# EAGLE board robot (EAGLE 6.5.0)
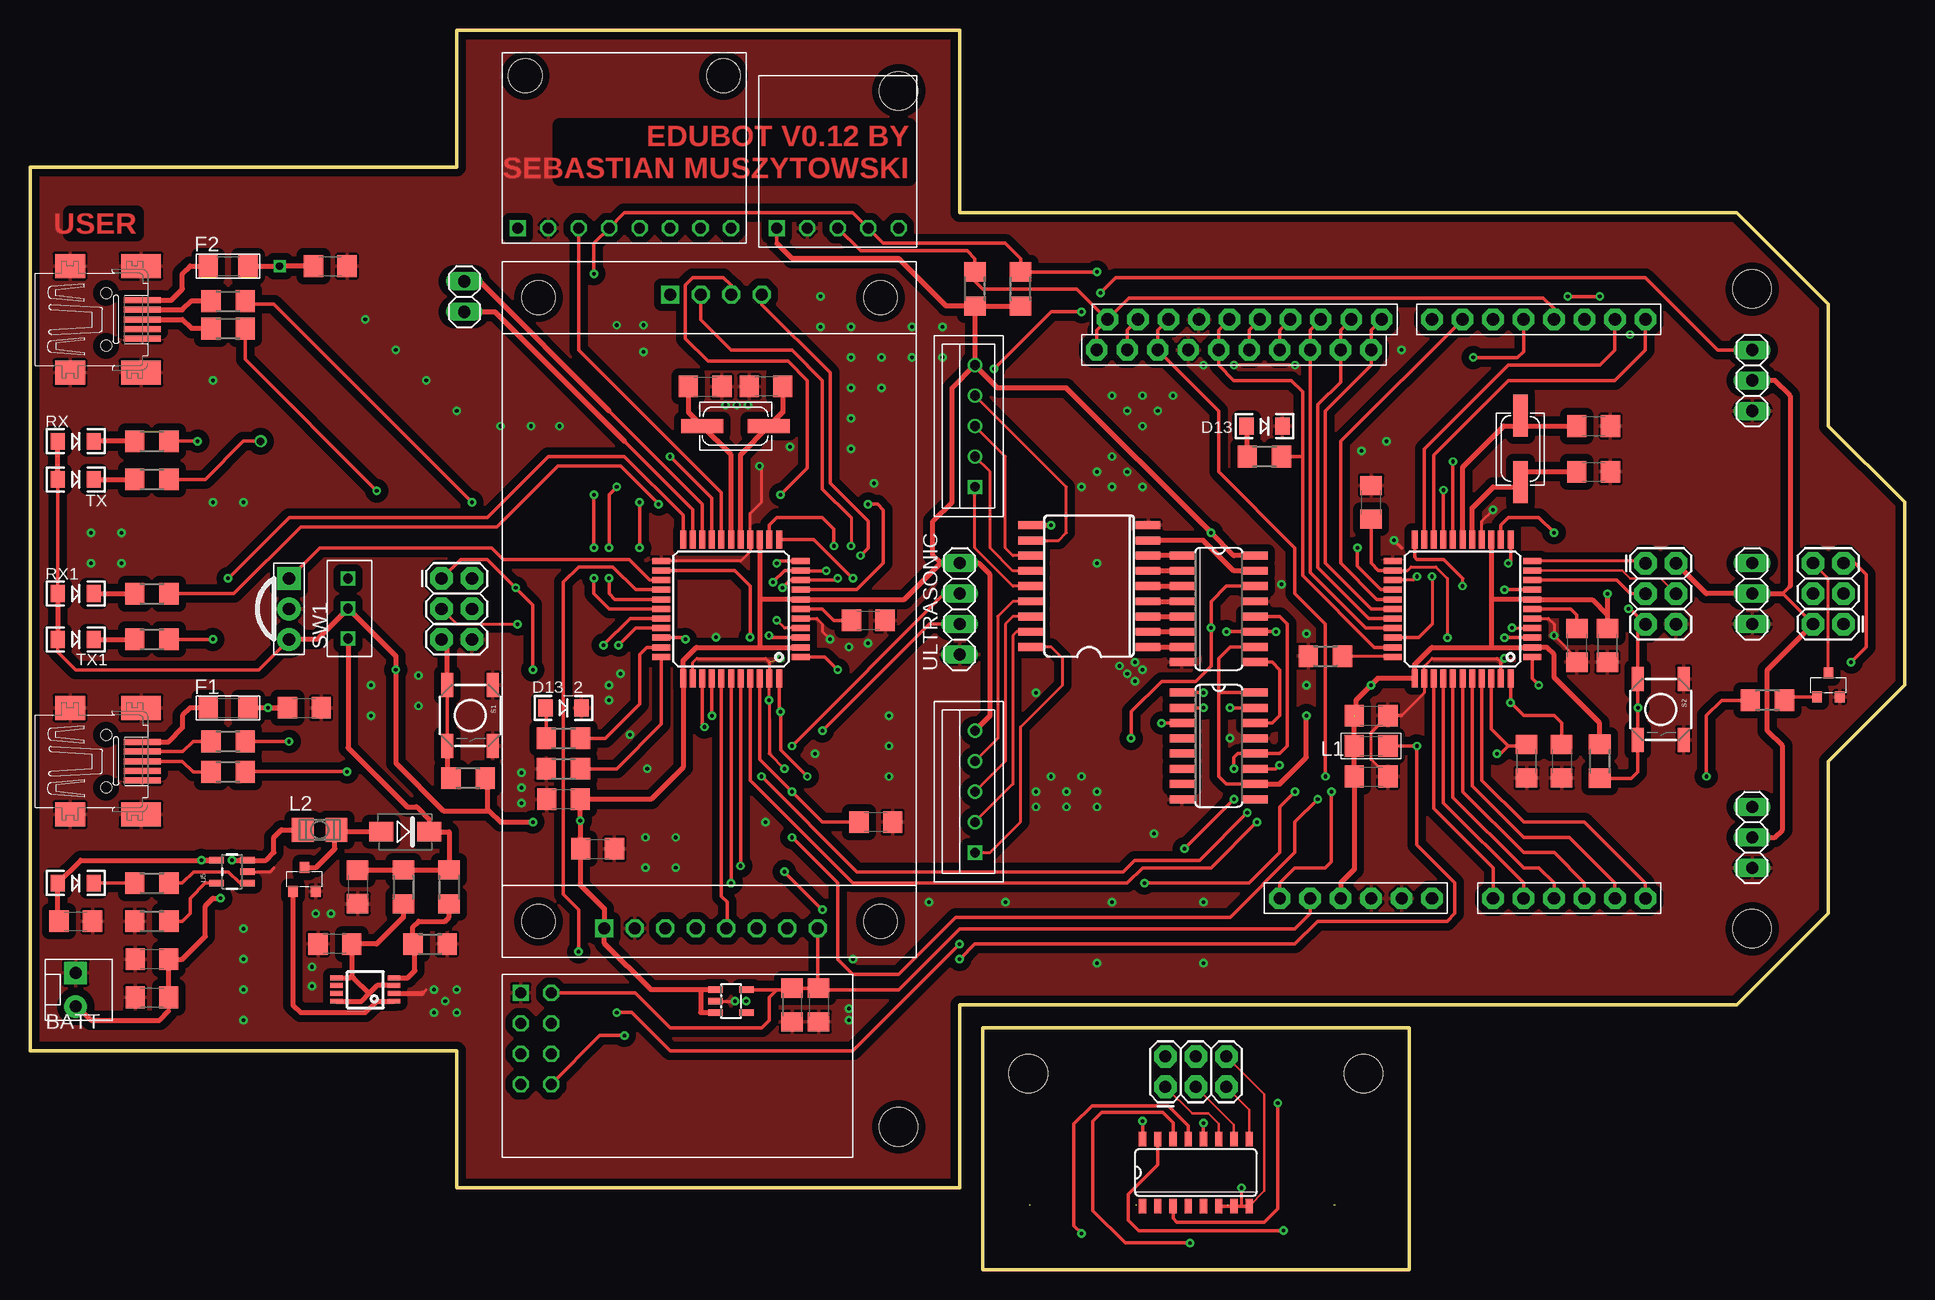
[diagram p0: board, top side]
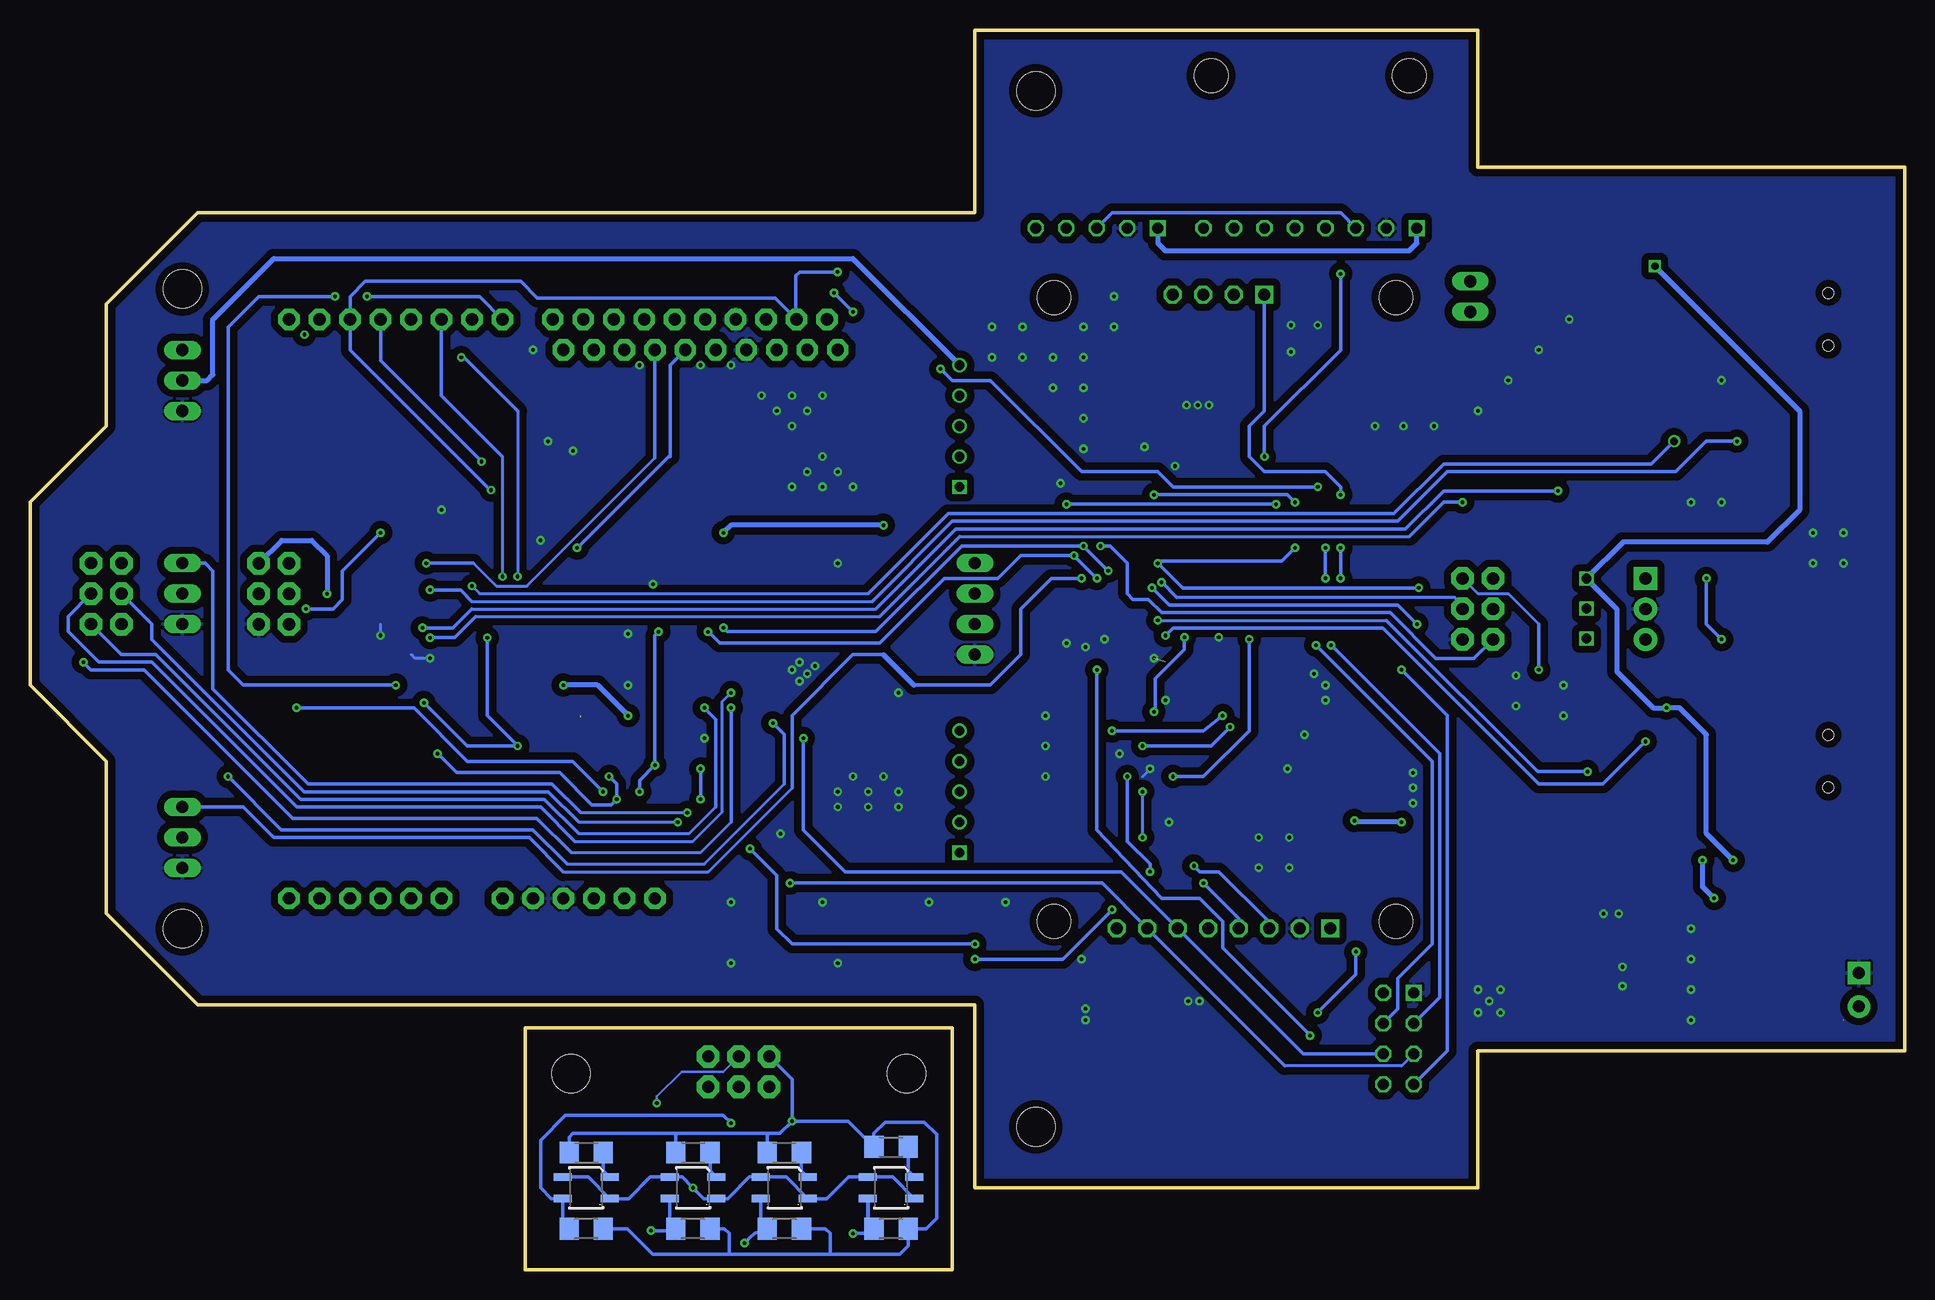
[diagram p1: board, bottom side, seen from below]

Size 156.21 x 103.35 mm. Coordinates in mm from the lower left corner, seen from the top.
Outline: 79.38,20.16 114.94,20.16 114.94,0 79.38,0 79.38,20.16
Outline: 156.21,48.74 149.86,42.39 149.86,29.69 142.24,22.07 77.47,22.07 77.47,6.83 35.56,6.83 35.56,18.26 0,18.26 0,91.92 35.56,91.92 35.56,103.35 77.47,103.35 77.47,88.11 142.24,88.11 149.86,80.49 149.86,70.33 156.21,63.98 156.21,48.74
Copper layers (1*16): Top 0.035mm / dielectric 1.5mm / Bottom 0.035mm
Design rules "pcb-devboards_35µmCU_200µm_Strukturen_Abstaende": minimum track width 0.2mm, minimum drill 0.3mm, track to track 0.2mm, track to pad 0.2mm, pad to pad 0.2mm, via to via 0.2mm, smd to smd 0.2mm, copper to edge 0.4mm, drill to drill 0.4mm, minimum pad ring 0.2mm, minimum via ring 0.2mm, stop-mask expansion 4mil, vias tented up to drill 0mil, thermal gap 0.2mm
Net classes: 1 vcc: width 0.254 mm
Holes 3.2 mm at 83.19,16.35 111.12,16.35 72.39,11.91 72.39,98.27 143.51,81.76 143.51,28.42

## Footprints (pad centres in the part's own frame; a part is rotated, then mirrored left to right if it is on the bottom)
MOLEX-1X2_LOCK = drill 1.016 pad 1.88 square: 1 -0.127,0 | drill 1.016 pad 1.88: 2 2.667,0
C1206 = smd 1.6 x 1.8: 1 -1.4,0; 2 1.4,0
1X06-BIG = drill 1.016 pad 1.778 octagon: 1 -6.35,0; 2 -3.81,0; 3 -1.27,0; 4 1.27,0; 5 3.81,0; 6 6.35,0
1X08-BIG = drill 1.016 pad 1.778 octagon: 1 -8.89,0; 2 -6.35,0; 3 -3.81,0; 4 -1.27,0; 5 1.27,0; 6 3.81,0; 7 6.35,0; 8 8.89,0
1X10-BIG = drill 1.016 pad 1.778 octagon: 1 -11.43,0; 2 -8.89,0; 3 -6.35,0; 4 -3.81,0; 5 -1.27,0; 6 1.27,0; 7 3.81,0; 8 6.35,0; 9 8.89,0; 10 11.43,0
SMA = smd 2 x 1.65: A 5,0.8; C 1,0.8
LED-1206 = smd 1.2 x 1.4: A -1.5,0; C 1.5,0
1206_PTC = smd 1.6 x 1.8: 1 -1.654,0; 2 1.654,0
MICRO3 = smd 0.8 x 0.9: 1 -0.95,-1; 2 0.95,-1; 3 0,1
2X3 = drill 1.016 pad 1.88 octagon: 1 0,0; 2 0,2.54; 3 2.54,0; 4 2.54,2.54; 5 5.08,0; 6 5.08,2.54
1206W = smd 1.6 x 1.8: 1 -1.4,0; 2 1.4,0
L3225P = smd 1.8 x 2: 1 -1.4,0; 2 1.4,0
32005-201 = smd 3.1 x 0.5: 1 3,1.6; 2 3,0.8; 3 3,0; 4 3,-0.8; 5 3,-1.6 | smd 2.5 x 2: M1 -3,-4.45; M2 -3,4.45 | smd 3.3 x 2: M3 2.9,4.45; M4 2.9,-4.45 | hole 0.9: 0,2.2; 0,-2.2
SO16 = smd 0.6 x 1.2: 1 -4.445,-2.8; 2 -3.175,-2.8; 3 -1.905,-2.8; 4 -0.635,-2.8; 5 0.635,-2.8; 6 1.905,-2.8; 7 3.175,-2.8; 8 4.445,-2.8; 9 4.445,2.8; 10 3.175,2.8; 11 1.905,2.8; 12 0.635,2.8; 13 -0.635,2.8; 14 -1.905,2.8; 15 -3.175,2.8; 16 -4.445,2.8
CSM-3X = smd 3.5 x 1.2: 1 2.775,0; 2 -2.775,0
QRE1113 = smd 1.5 x 0.6: 1 -1.95,-0.9; 2 1.95,-0.9; 3 1.95,0.9; 4 -1.95,0.9
R1206 = smd 1.6 x 1.803: 1 -1.422,0; 2 1.422,0
TACTILE_SWITCH_SMD = smd 2 x 1: 1 -2.54,1.905; 2 2.54,1.905; 3 -2.54,-1.905; 4 2.54,-1.905
1X02 = drill 1.016 long: 1 -1.27,0; 2 1.27,0
1X03 = drill 1.016 long: 1 -2.54,0; 2 0,0; 3 2.54,0
SO16' = smd 0.66 x 2.032: 1 -4.445,-3.073; 2 -3.175,-3.073; 3 -1.905,-3.073; 4 -0.635,-3.073; 5 0.635,-3.073; 6 1.905,-3.073; 7 3.175,-3.073; 8 4.445,-3.073; 9 4.445,3.073; 10 3.175,3.073; 11 1.905,3.073; 12 0.635,3.073; 13 -0.635,3.073; 14 -1.905,3.073; 15 -3.175,3.073; 16 -4.445,3.073
SO18L = smd 0.66 x 2.032: 1 -0.635,-4.902; 2 0.635,-4.902; 3 1.905,-4.902; 4 3.175,-4.902; 5 4.445,-4.902; 6 5.715,-4.902; 7 6.985,-4.902; 8 8.255,-4.902; 9 9.525,-4.902; 10 9.525,4.902; 11 8.255,4.902; 12 6.985,4.902; 13 5.715,4.902; 14 4.445,4.902; 15 3.175,4.902; 16 1.905,4.902; 17 0.635,4.902; 18 -0.635,4.902
SPDT-PTH = drill 0.8 square: 1 1.5,-1.75; 2 4,-1.75; 3 6.5,-1.75
TQFP44 = smd 1.5 x 0.5: 1 -5.8,4; 2 -5.8,3.2; 3 -5.8,2.4; 4 -5.8,1.6; 5 -5.8,0.8; 6 -5.8,0; 7 -5.8,-0.8; 8 -5.8,-1.6; 9 -5.8,-2.4; 10 -5.8,-3.2; 11 -5.8,-4; 23 5.8,-4; 24 5.8,-3.2; 25 5.8,-2.4; 26 5.8,-1.6; 27 5.8,-0.8; 28 5.8,0; 29 5.8,0.8; 30 5.8,1.6; 31 5.8,2.4; 32 5.8,3.2; 33 5.8,4 | smd 0.5 x 1.5: 12 -4,-5.8; 13 -3.2,-5.8; 14 -2.4,-5.8; 15 -1.6,-5.8; 16 -0.8,-5.8; 17 0,-5.8; 18 0.8,-5.8; 19 1.6,-5.8; 20 2.4,-5.8; 21 3.2,-5.8; 22 4,-5.8; 34 4,5.8; 35 3.2,5.8; 36 2.4,5.8; 37 1.6,5.8; 38 0.8,5.8; 39 0,5.8; 40 -0.8,5.8; 41 -1.6,5.8; 42 -2.4,5.8; 43 -3.2,5.8; 44 -4,5.8
SOT23-5@1 = smd 0.55 x 1.2: 1 -0.95,-1.3; 2 0,-1.3; 3 0.95,-1.3; 4 0.95,1.3; 5 -0.95,1.3
MSOP8 = smd 0.41 x 1.02: 1 -0.95,-2.4; 2 -0.3,-2.4; 3 0.35,-2.4; 4 1,-2.4; 5 1,2.4; 6 0.35,2.4; 7 -0.3,2.4; 8 -0.95,2.4
SOT23-5 = smd 0.55 x 1.2: 1 -0.95,-1.3; 2 0,-1.3; 3 0.95,-1.3; 4 0.95,1.3; 5 -0.95,1.3
1.8TFTSD = drill 1 square: P$1 55.58,8.5; P$9 2.76,14 | drill 1 octagon: P$2 55.58,11.04; P$3 55.58,13.58; P$4 55.58,16.12; P$5 55.58,18.66; P$6 55.58,21.2; P$7 55.58,23.74; P$8 55.58,26.28; P$10 2.76,16.54; P$11 2.76,19.08; P$12 2.76,21.62 | hole 2.8: 3,3; 3,31.5; 55,31.5; 55,3
GY-521 = drill 0.9 square: P$1 0,0 | drill 0.9 octagon: P$2 2.54,0; P$3 5.08,0; P$4 7.62,0; P$5 10.16,0; P$6 12.7,0; P$7 15.24,0; P$8 17.78,0 | hole 2.8: 0.635,12.7; 17.145,12.7
HMC5883L = drill 0.9 square: P$1 0,5.08 | drill 0.9 octagon: P$2 0,2.54; P$3 0,0; P$4 0,-2.54; P$5 0,-5.08
NRF24L01+ = drill 0.9 square: P$1 -1.016,1.016 | drill 0.9 octagon: P$2 -1.016,-1.524; P$3 -1.016,-4.064; P$4 -1.016,-6.604; P$5 1.524,-6.604; P$6 1.524,-4.064; P$7 1.524,-1.524; P$8 1.524,1.016
PNA460XM = drill 1.016 pad 1.93 square: 1 -2.54,0 | drill 1.016 pad 1.93: 2 0,0; 3 2.54,0
1X04 = drill 1.016 long: 1 -3.81,0; 2 -1.27,0; 3 1.27,0; 4 3.81,0
B5B-XH = drill 0.8 square: P$1 -5.08,0 | drill 0.8: P$2 -2.54,0; P$3 0,0; P$4 2.54,0; P$5 5.08,0

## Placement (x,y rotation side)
BATT  M02POLAR_LOCK  [MOLEX-1X2_LOCK]  3.81,24.61 270 top
C1  0.1uF  [C1206]  124.71,42.39 90 top
C2  0.1uF  [C1206]  44.45,39.21 180 top
C3  1uF  [C1206]  128.91,52.04 270 top
C4  1uF  [C1206]  131.44,52.04 270 top
C5  10uF  [C1206]  22.86,46.83 0 top
C6  10uF  [C1206]  25.02,83.66 0 top
C7  10uF  [C1206]  63.5,22.07 270 top
C8  0.1uF  [C1206]  70.48,37.31 180 top
C9  1uF  [C1206]  69.85,54.13 0 top
C10  0.1uF  [C1206]  111.76,46.2 0 top
C11  100nF  [C1206]  65.72,22.07 270 top
C12  1uF  [C1206]  111.76,41.12 0 top
C13  0.1uF  [C1206]  111.76,63.98 90 top
C14  0.1uF  [C1206]  127.64,42.39 270 top
C15  18pF  [C1206]  130.3,70.33 0 top
C16  18pF  [C1206]  130.3,66.52 0 top
C17  1uF  [C1206]  47.31,35.08 0 top
C18  47 uF  [C1206]  10.16,22.7 0 top
C19  0.1uF  [C1206]  25.4,27.15 180 top
C20  4.7uF  [C1206]  3.81,29.05 0 top
C21  4.7uF  [C1206]  10.16,25.88 180 top
C22  18pF  [C1206]  56.26,73.63 0 top
C23  18pF  [C1206]  61.34,73.63 180 top
C24  47 uF  [C1206]  27.3,31.91 270 top
CONN1  ANALOG  [1X06-BIG]  128.27,30.96 0 top
CONN2  DIGITAL  [1X08-BIG]  125.73,79.22 180 top
CONN3  DIGITAL  [1X10-BIG]  101.22,79.22 180 top
CONN4  DIGITAL RASTER  [1X10-BIG]  100.33,76.68 180 top
CONN5  POWER  [1X06-BIG]  110.49,30.96 0 top
D3  B330A  [SMA]  34.29,37.31 180 top
D4  POWER  [LED-1206]  3.81,32.23 0 top
D13  Green  [LED-1206]  102.87,70.33 0 top
D13_2  Green  [LED-1206]  44.45,46.83 0 top
F1  1206L  [1206_PTC]  16.51,46.83 0 top
F2  1206L  [1206_PTC]  16.51,83.66 0 top
FET1  TR  [MICRO3]  149.86,48.74 0 top
FET3  TR  [MICRO3]  22.86,32.54 0 top
JP1  ISP  [2X3]  34.29,57.63 270 top
JP2  [2X3]  151.13,53.82 90 top
JP3  ISP  [2X3]  134.62,58.89 270 top
JP4  [2X3]  94.61,15.24 0 top
L1  Ferrite  [1206W]  111.76,43.66 0 top
L2  BRL3225T3R3M  [L3225P]  24.13,36.67 0 top
MINIUSB  MINI-USB-SCHIELD-32005-201  [32005-201]  6.35,79.22 0 top
MINIUSB1  MINI-USB-SCHIELD-32005-201  [32005-201]  6.35,42.39 0 top
MUX  74HC4051  [SO16]  97.16,8.1 0 top
Q1  CSM-3X-CRYSTALCSM-3X  [CSM-3X]  124.21,68.42 90 top
Q2  QRE1113  [QRE1113]  84.45,6.83 180 bottom
Q3  QRE1113  [QRE1113]  93.34,6.83 180 bottom
Q4  QRE1113  [QRE1113]  100.97,6.83 180 bottom
Q5  QRE1113  [QRE1113]  109.86,6.83 180 bottom
Q6  CSM-3X-CRYSTALCSM-3X  [CSM-3X]  58.8,70.33 180 top
R1  100  [R1206]  84.45,10.24 180 bottom
R2  10K  [R1206]  130.81,42.39 90 top
R3  10K  [R1206]  84.45,3.41 0 bottom
R4  22  [R1206]  16.51,78.45 180 top
R5  22  [R1206]  16.51,80.74 180 top
R6  1K  [R1206]  102.87,67.79 180 top
R7  1K  [R1206]  10.16,69.06 180 top
R8  1K  [R1206]  10.16,65.88 180 top
R9  10K  [R1206]  107.95,51.15 180 top
R10  100  [R1206]  93.34,9.76 180 bottom
R11  10K  [R1206]  93.34,3.41 0 bottom
R12  100  [R1206]  100.97,9.76 180 bottom
R13  10K  [R1206]  100.97,3.41 0 bottom
R14  100  [R1206]  109.86,9.76 180 bottom
R15  10K  [R1206]  109.86,3.41 0 bottom
R16  22  [R1206]  16.51,41.5 180 top
R17  470  [R1206]  10.16,32.23 180 top
R18  100  [R1206]  144.78,47.47 0 top
R19  2K  [R1206]  10.16,29.05 180 top
R20  1K  [R1206]  44.45,44.29 180 top
R21  1K  [R1206]  10.16,56.36 180 top
R22  1K  [R1206]  10.16,52.55 180 top
R23  10K  [R1206]  36.51,40.96 0 top
R24  10K  [R1206]  44.45,41.75 180 top
R25  22  [R1206]  16.51,44.04 180 top
R26  2.2K  [R1206]  78.74,81.76 270 top
R27  2.2K  [R1206]  82.55,81.76 270 top
R46  100  [R1206]  31.11,31.91 90 top
R49  3.09k  [R1206]  34.92,31.91 90 top
R51  1K  [R1206]  33.34,27.15 180 top
RX  Green  [LED-1206]  3.81,69.06 0 top
RX1  Green  [LED-1206]  3.81,56.36 0 top
S1  Reset  [TACTILE_SWITCH_SMD]  36.67,46.2 270 top
S2  Reset  [TACTILE_SWITCH_SMD]  135.89,46.7 270 top
SER_CPU2  SER2  [1X02]  36.2,81.12 90 top
SERVO1(USONIC)  USONIC  [1X03]  143.51,56.36 90 top
SERVO2(GRIP)  GRIPPER  [1X03]  143.51,74.14 90 top
SERVO3(GRIPROT)  ROTATE  [1X03]  143.51,36.04 90 top
SHIFT1  74HC595D  [SO16']  99.06,55.09 270 top
SHIFT2  74HC595D  [SO16']  99.06,43.66 270 top
STEPPER_DRIVER  ULN2803  [SO18L]  88.27,52.55 90 top
SW1  [SPDT-PTH]  24.77,51.12 90 top
TX  Green  [LED-1206]  3.81,65.88 0 top
TX1  Green  [LED-1206]  3.81,52.55 0 top
U1  USER  [TQFP44]  119.38,55.09 180 top
U2  BRAIN  [TQFP44]  58.42,55.09 180 top
U3  LP2985  [SOT23-5@1]  58.42,22.38 270 top
U4  MCP1650  [MSOP8]  27.94,23.34 90 top
U5  MCP73831  [SOT23-5]  16.83,33.18 90 top
U$2  1.8TFT+SD  [1.8TFTSD]  39.37,84.04 270 top
U$3  GY-521  [GY-521]  40.64,86.84 0 top
U$4  HMC5883L  [HMC5883L]  67.31,86.84 90 top
U$5  NRF24L01+  [NRF24L01+]  41.91,22.07 0 top
U$10  PNA460XM  [PNA460XM]  21.59,55.09 270 top
ULTRASONIC  [1X04]  77.47,55.09 90 top
X1  05-JST-B5B-XH-A  [B5B-XH]  78.74,39.85 90 top
X2  05-JST-B5B-XH-A  [B5B-XH]  78.74,70.33 90 top

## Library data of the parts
BATT JP2 JP4 = SparkFun-Connectors
C1-C24 L2 R1-R27 R46 R49 R51 = resistor
CONN1-CONN5 U1 U2 U$10 = adafruit
D3 FET1 FET3 Q2-Q5 = aaron_discrete
D4 D13 D13_2 RX RX1 TX TX1 = SparkFun-LED
F1 F2 = microbuilder
JP1 JP3 S1 S2 U3 U5 = SparkFun
L1 = wuerth-elektronik
MINIUSB MINIUSB1 = con-cypressindustries; OC_FARNELL: unknown; OC_NEWARK: unknown
MUX = SparkFun-AnalogIC
Q1 Q6 = fmc
SER_CPU2 SERVO1(USONIC) SERVO2(GRIP) SERVO3(GRIPROT) ULTRASONIC = pinhead
SHIFT1 SHIFT2 = 74xx-eu
STEPPER_DRIVER = SparkFun-PowerIC
SW1 = switch
U4 = aaron_ic
U$2-U$5 = muzy_robot
X1 X2 = con-jst-xh

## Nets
2D13: R20.1 U2.32
2D+: R16.1 U2.4
2D-: R25.1 U2.3
2MISO: JP1.1 U2.11 U$2.P$11 U$5.P$4
2MOSI: JP1.4 SHIFT1.14 U2.10 U$2.P$6 U$2.P$10 U$5.P$6
2RESET: JP1.5 R23.1 S1.3 S1.4 U2.13
2RXLED: R21.1 U2.8
2SCK: JP1.3 SHIFT1.11 SHIFT2.11 U2.9 U$2.P$7 U$2.P$12 U$5.P$3
2TXLED: R22.1 U2.22
2XTAL1: C22.1 Q6.1 U2.17
2XTAL2: C23.1 Q6.2 U2.16
3.3V: C7.1 C11.1 CONN5.2 U3.5 U$2.P$8 U$5.P$8
A0: CONN1.1 U1.36
A1: CONN1.2 U1.37
A2: CONN1.3 U1.38
A3: CONN1.4 U1.39
A4: CONN1.5 U1.40
A5: CONN1.6 U1.41
AREF: C1.2 C8.2 CONN3.8 CONN4.8 U1.42 U2.42
AVCC: C13.1 C14.1 L1.2 U1.24 U1.44 U2.24 U2.44
BATT_OUT: C24.1 D3.C R46.2 R49.2 SW1.1
D4: CONN2.5 U1.25
D5: CONN2.6 U1.31
D6: CONN2.7 U1.27
D7: CONN2.8 U1.1
D8: CONN3.1 CONN4.1 U1.28
D9: CONN3.2 CONN4.2 U1.29
D10: CONN3.3 CONN4.3 U1.30
D11: CONN3.4 CONN4.4 U1.12
D12: CONN3.5 CONN4.5 U1.26
D13: CONN3.6 CONN4.6 R6.1 U1.32
D+: R4.1 U1.4
D-: R5.1 U1.3
ECHO: U2.37 ULTRASONIC.2
GND: BATT.1 C1.1 C2.2 C3.2 C4.2 C5.2 C6.2 C7.2 C8.1 C9.2 C10.2 C11.2 C12.2 C13.2 C14.2 C15.2 C16.2 C17.2 C18.1 C19.2 C20.2 C21.2 C22.2 C23.2 C24.2 CONN3.7 CONN4.7 CONN5.4 CONN5.5 D13.C D13_2.C FET1.2 FET3.2 JP1.6 JP3.6 MINIUSB1.5 MINIUSB1.M1 MINIUSB1.M2 MINIUSB1.M3 MINIUSB1.M4 MINIUSB.5 MINIUSB.M1 MINIUSB.M2 MINIUSB.M3 MINIUSB.M4 R9.2 R19.2 R24.2 R51.1 S1.1 S1.2 S2.1 S2.2 SERVO1(USONIC).1 SERVO2(GRIP).1 SERVO3(GRIPROT).1 SHIFT1.8 SHIFT1.13 SHIFT2.8 SHIFT2.13 STEPPER_DRIVER.9 U1.5 U1.15 U1.23 U1.35 U1.43 U2.5 U2.15 U2.23 U2.35 U2.43 U3.2 U4.2 U5.2 U$2.P$2 U$3.P$2 U$4.P$2 U$5.P$1 U$10.2 ULTRASONIC.1
IR: U2.25 U$10.1
IR_GND: JP4.6 MUX.6 MUX.7 MUX.8 Q2.2 Q2.4 Q3.2 Q3.4 Q4.2 Q4.4 Q5.2 Q5.4
IR_OUT: JP4.4 MUX.3
IR_VCC: JP4.2 MUX.16 R1.2 R3.2 R10.2 R11.2 R12.2 R13.2 R14.2 R15.2
IRA: JP4.1 MUX.11
IRB: JP4.3 MUX.10
IRC: JP4.5 MUX.9
MISO: JP3.1 U1.11
MOSI: JP3.4 U1.10
MUX0: MUX.13 Q2.3 R3.1
MUX1: MUX.14 Q3.3 R11.1
MUX2: MUX.15 Q4.3 R13.1
MUX3: MUX.12 Q5.3 R15.1
MUX_OUT: JP2.4 U2.41
N$1: R8.2 TX.C
N$2: MINIUSB.2 R5.2
N$3: SER_CPU2.1 U2.21
N$4: SER_CPU2.2 U2.20
N$5: MINIUSB.3 R4.2
N$6: R9.1 U1.33
N$7: D13.A R6.2
N$8: C9.1 U2.6
N$9: R7.2 RX.C
N$10: Q2.1 R1.1
N$11: Q3.1 R10.1
N$12: Q4.1 R12.1
N$13: F2.1 MINIUSB.1
N$14: Q5.1 R14.1
N$15: C3.1 U1.6
N$16: FET1.1 R18.2
N$17: R24.1 U2.33
N$18: F1.1 MINIUSB1.1
N$19: FET3.1 U4.1
N$20: R19.1 U5.5
N$21: R17.1 U5.1
N$22: D4.C R17.2
N$23: R49.1 R51.2 U4.4
N$24: D3.A FET3.3 L2.2
N$25: C19.1 R46.1 U4.3 U4.5 U4.8
N$26: STEPPER_DRIVER.11 X2.P$4
N$27: STEPPER_DRIVER.12 X2.P$3
N$28: STEPPER_DRIVER.13 X2.P$2
N$29: STEPPER_DRIVER.14 X2.P$1
N$30: STEPPER_DRIVER.15 X1.P$4
N$31: STEPPER_DRIVER.16 X1.P$3
N$32: STEPPER_DRIVER.17 X1.P$2
N$33: STEPPER_DRIVER.18 X1.P$1
N$34: D13_2.A R20.2
N$35: R22.2 TX1.C
N$36: R21.2 RX1.C
N$37: MINIUSB1.2 R25.2
N$38: MINIUSB1.3 R16.2
N$41: JP2.1 SHIFT2.15
N$42: JP2.3 SHIFT2.1
N$43: JP2.5 SHIFT2.2
N$45: FET1.3 JP2.6
NRF_CE: U2.29 U$5.P$2
NRF_CSN: U2.30 U$5.P$7
NRF_IRQ: U2.1 U$5.P$5
RESET: CONN5.1 JP3.5 R2.1 S2.3 S2.4 U1.13
RX-I: CONN2.1 U1.20
RXLED: R7.1 U1.8
S1: SHIFT1.15 STEPPER_DRIVER.8
S1OVERFLOW: SHIFT1.9 SHIFT2.14
S2: SHIFT1.1 STEPPER_DRIVER.7
S2O4: R18.1 SHIFT2.3
S3: SHIFT1.2 STEPPER_DRIVER.6
S4: SHIFT1.3 STEPPER_DRIVER.5
S5: SHIFT1.4 STEPPER_DRIVER.4
S6: SHIFT1.5 STEPPER_DRIVER.3
S7: SHIFT1.6 STEPPER_DRIVER.2
S8: SHIFT1.7 STEPPER_DRIVER.1
S_GRIP: SERVO2(GRIP).3 U2.27
S_GRIPROT: SERVO3(GRIPROT).3 U2.12
S_USONIC: SERVO1(USONIC).3 U2.31
SCK: JP3.3 U1.9
SCL: CONN2.4 CONN3.10 CONN4.10 R26.1 U1.18 U2.18 U$3.P$3 U$4.P$3
SD_CS: U2.28 U$2.P$9
SDA: CONN2.3 CONN3.9 CONN4.9 R27.1 U1.19 U2.19 U$3.P$4 U$4.P$4
SHIFT_RCK: SHIFT1.12 SHIFT2.12 U2.26
TFT_CS: U2.40 U$2.P$3
TFT_DC: U2.38 U$2.P$5
TFT_RST: U2.39 U$2.P$4
TRIG: U2.36 ULTRASONIC.3
TX-O: CONN2.2 U1.21
TXLED: R8.1 U1.22
USB_VIN: C5.1 C6.1 C20.1 D4.A F1.2 F2.2 SW1.3 U5.4
VBATT: BATT.2 C18.2 C21.1 L2.1 U5.3
VCC: C2.1 C4.1 C10.1 C12.1 C17.1 CONN5.3 JP1.2 JP2.2 JP3.2 L1.1 R2.2 R23.2 R26.2 R27.2 RX1.A RX.A SERVO1(USONIC).2 SERVO2(GRIP).2 SERVO3(GRIPROT).2 SHIFT1.10 SHIFT1.16 SHIFT2.10 SHIFT2.16 STEPPER_DRIVER.10 SW1.2 TX1.A TX.A U1.2 U1.7 U1.14 U1.34 U2.2 U2.7 U2.14 U2.34 U3.1 U3.3 U$2.P$1 U$3.P$1 U$4.P$1 U$10.3 ULTRASONIC.4 X1.P$5 X2.P$5
XTAL1: C15.1 Q1.1 U1.17
XTAL2: C16.1 Q1.2 U1.16

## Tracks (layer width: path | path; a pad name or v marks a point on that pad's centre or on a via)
2D13
  Top 0.305: 52.59,51.91 U2.32 51.41,51.89 50.8,51.28 50.8,47.15 47.94,44.29 R20.1
2D+  (via drill 0.3 pad 0.3)
  Top 0.254: U2.4 62.88,53.49 v62.23,54.13
  Top 0.305: v26.43,41.51 17.95,41.51 R16.1
  Bottom 0.254: v62.23,54.13 43.18,54.13
  Bottom 0.305: 43.18,54.13 30.56,41.51 v26.43,41.51
2D-  (via drill 0.3 pad 0.3)
  Top 0.305: U2.3 61.77,52.69 v61.59,52.86 | R25.1 v21.59,44.04
  Bottom 0.305: v61.59,52.86 60.96,53.5 43.5,53.5 30.48,40.48 25.15,40.48 v21.59,44.04
2MISO  (via drill 0.3 pad 0.3)
  Top 0.305: v50.8,60.17 v50.8,63.98 | v62.55,64.61 64.77,66.83 64.77,74.14 63.18,75.72 56.52,75.72 54.61,77.63 54.61,82.07 55.24,82.71 57.78,82.71 58.42,82.07 58.42,81.28 U$2.P$11 | v62.23,58.9 62.42,59.09 U2.11 | JP1.1 35.88,59.21 38.1,59.21 v40.48,56.83 41.91,55.4 v41.91,50.01
  Bottom 0.305: v40.48,56.83 60.17,56.83 v62.23,58.9 62.04,59.09 51.88,59.09 v50.8,60.17 | v50.8,63.98 51.44,64.61 v62.55,64.61 | U$5.P$4 38.1,18.26 38.1,46.2 v41.91,50.01
2MOSI  (via drill 0.3 pad 0.3)
  Top 0.254: 68.42,62.71 v68.42,60.33
  Top 0.305: v61.91,57.31 62.89,58.29 U2.10 64.25,58.26 v66.36,58.26 | SHIFT1.14 99.69,56.99 98.42,55.72 v98.42,53.5 98.42,50.32 97.16,49.05 94.3,49.05 91.76,46.51 v91.76,44.29 | U$2.P$10 55.91,79.19 58.42,76.68 63.5,76.68 66.04,74.14 66.04,65.09 68.42,62.71
  Bottom 0.254: JP1.4 37.47,56.04 60.64,56.04
  Bottom 0.305: U$5.P$6 50.11,18 U$2.P$6 65.29,33.18 88.27,33.18 91.76,36.67 v91.76,44.29 | 60.64,56.04 v61.91,57.31 | v98.42,53.5 98.11,53.18 85.72,53.18 78.58,60.33 v68.42,60.33 v66.36,58.26
2RESET  (via drill 0.3 pad 0.3)
  Top 0.305: S1.3 S1.4 | U2.13 61.62,62.1 62.23,62.71 66.04,62.71 66.99,61.75 v66.99,60.33
  Top 0.406: S1.3 34.77,52.07 JP1.5 | S1.4 34.77,41.28 R23.1
  Bottom 0.305: v66.99,60.33 66.2,60.33 64.77,58.9 64.77,56.36 64.29,55.88 63.02,55.88 61.91,54.77 42.86,54.77 39.05,50.96 35.88,50.96 JP1.5
2RXLED  (via drill 0.3 pad 0.3)
  Top 0.305: U2.8 68.91,56.69 71.12,58.9 71.12,63.34 70.64,63.82 v69.85,63.82 | v52.39,63.82 49.21,66.99 43.97,66.99 38.89,61.91 22.54,61.91 16.99,56.36 R21.1
  Bottom 0.305: v69.85,63.82 v52.39,63.82
2SCK  (via drill 0.3 pad 0.3)
  Top 0.254: JP1.3 35.56,53.82 v40.64,53.82
  Top 0.305: SHIFT2.11 103.82,41.75 v104.14,42.07 | v103.82,53.18 SHIFT1.11 v99.69,53.18 | v62.71,56.83 63.36,57.49 U2.9 67.17,57.49 v67.31,57.63 | v92.87,32.23 101.6,32.23 104.14,34.77 104.14,38.58 v105.41,39.85 | U$2.P$12 60.99,80.46 66.67,74.77 66.67,65.56 69.85,62.39 69.85,60.17 v69.22,59.53
  Bottom 0.254: U$5.P$3 41.91,16.99 51.63,16.99
  Bottom 0.305: 51.63,16.99 U$2.P$7 66.87,32.23 v92.87,32.23 | v103.82,53.18 104.14,52.86 v104.14,42.07 105.41,40.8 v105.41,39.85 | v40.64,53.82 42.23,55.4 61.28,55.4 v62.71,56.83 | v67.31,57.63 v69.22,59.53 73.66,59.53 75.56,57.63 80.01,57.63 85.41,52.23 98.74,52.23 v99.69,53.18
2TXLED  (via drill 0.3 pad 0.3)
  Top 0.305: U2.22 54.42,62.9 49.53,67.79 43.18,67.79 38.1,62.71 21.59,62.71 v16.51,57.63 | v15.24,52.55 R22.1
  Bottom 0.305: v16.51,57.63 16.51,53.82 v15.24,52.55
2XTAL1
  Top 0.406: C22.1 54.86,71.49 Q6.1 58.42,67.93 U2.17
2XTAL2
  Top 0.406: C23.1 62.74,71.49 Q6.2 59.22,67.97 U2.16
3.3V
  Top 0.305: C11.1 C7.1 63.37,23.33 62.23,23.33 | U$2.P$8 65.65,23.47 C11.1 | CONN5.2 106.68,29.69 105.41,28.42 77.47,28.42 72.39,23.34 65.85,23.34 C11.1 | 62.23,23.33 U3.5 | U$5.P$8 50.42,23.08 53.34,20.16 60.96,20.16 61.59,20.8 61.59,22.7 62.23,23.33
A0
  Top 0.305: U1.36 116.98,38.44 121.92,33.5 CONN1.1
A1
  Top 0.305: U1.37 117.78,38.91 124.46,32.23 CONN1.2
A2
  Top 0.305: U1.38 118.58,39.38 124.46,33.5 125.73,33.5 127,32.23 CONN1.3
A3
  Top 0.305: U1.39 119.38,39.85 124.46,34.77 127,34.77 129.54,32.23 CONN1.4
A4
  Top 0.305: U1.40 120.18,40.32 124.46,36.04 128.27,36.04 132.08,32.23 CONN1.5
A5
  Top 0.305: U1.41 120.98,40.79 124.46,37.31 129.54,37.31 134.62,32.23 CONN1.6
AREF  (via drill 0.3 pad 0.3)
  Top 0.305: U1.42 121.78,45.07 123.19,43.66 | 123.19,43.66 124.58,43.66 C1.2 | CONN3.8 93.98,78.33 CONN4.8 99.06,71.6 99.06,66.52 105.41,60.17 105.41,56.36 107.95,53.82 v107.95,41.12 | v122.24,43.02 122.56,43.02 123.19,43.66 | U2.42 60.82,42.53 v63.5,39.85 66.04,37.31 C8.2 | v107.31,39.21 105.41,37.31 105.41,34.77 100.01,29.37 77.15,29.37 72.39,24.61 68.58,24.61 67.31,25.88 67.31,32.23 v63.5,36.04
  Bottom 0.254: v63.5,36.04 v63.5,39.85
  Bottom 0.305: v107.95,41.12 107.31,40.48 v107.31,39.21 107.79,38.74 109.38,38.74 112.08,41.43 120.65,41.43 v122.24,43.02
AVCC  (via drill 0.3 pad 0.3)
  Top 0.254: U1.24 114.8,58.29 115.09,58.58 117.16,58.58 118.11,57.63 v118.11,52.67
  Top 0.305: U1.44 v123.38,47.28 124.46,46.2 127,46.2 127.64,45.56 C14.1 | U1.24 112.37,58.29 111.76,58.9 C13.1 | U2.24 58.71,58.29 60.01,56.99 v60.01,52.71 | U2.44 62.42,46.7 v62.55,46.51 62.55,43.34 v64.77,41.12 | L1.2 v115.57,43.66 115.57,35.4 118.75,32.23 118.75,29.69 118.11,29.05 107.31,29.05 105.41,27.15 78.74,27.15 v77.47,25.88 | v66.04,30 v62.87,33.18
  Bottom 0.305: v123.38,47.28 119.76,43.66 v115.57,43.66 118.11,46.2 v118.11,52.67 | v60.01,52.71 60.01,51.7 U2.44 62.42,46.7 v62.55,46.51 | v77.47,25.88 70.17,25.88 v66.04,30 | v62.87,33.18 62.87,33.81 64.77,35.72 v64.77,41.12
BATT_OUT
  Top 0.406: R46.2 R49.2 | R49.2 34.92,36.51 D3.C 33.29,37.51 32.23,38.58 31.43,38.58 26.52,43.49 SW1.1 | C24.1 34.92,33.34 R49.2
D4  (via drill 0.3 pad 0.3)
  Top 0.254: v115.57,57.79 115.27,57.49 U1.25
  Top 0.305: CONN2.5 124.46,76.55 123.95,76.04 v120.27,76.04
  Bottom 0.254: 115.57,71.6 v115.57,57.79
  Bottom 0.305: v120.27,76.04 120.02,76.04 115.57,71.6
D5  (via drill 0.3 pad 0.3)
  Top 0.254: v116.84,57.79 116.84,53.82
  Top 0.305: U1.31 115.71,52.69 116.84,53.82
  Bottom 0.254: 116.84,67.79 v116.84,57.79
  Bottom 0.305: CONN2.6 121.92,72.87 116.84,67.79
D6
  Top 0.305: U1.27 112.23,55.89 109.22,58.9 109.22,69.06 CONN2.7
D7  (via drill 0.3 pad 0.3)
  Top 0.305: U1.1 125.18,49.29 v125.73,48.74 | v130.81,81.12 v128.14,81.12
  Bottom 0.305: v125.73,48.74 138.43,48.74 139.7,50.01 139.7,78.58 137.16,81.12 v130.81,81.12 | v128.14,81.12 118.75,81.12 CONN2.8
D8
  Top 0.305: CONN3.1 111.76,78.33 CONN4.1 111.76,75.41 107.95,71.6 107.95,58.9 111.76,55.09 U1.28
D9
  Top 0.305: CONN3.2 109.22,78.33 CONN4.2 109.22,74.01 107.31,72.1 107.31,58.52 111.54,54.29 U1.29
D10
  Top 0.305: CONN3.3 106.68,78.33 CONN4.3 106.68,58.13 111.33,53.49 U1.30
D11  (via drill 0.3 pad 0.3)
  Top 0.305: CONN4.4 104.14,78.33 CONN3.4 | U1.12 123.38,59.09 v123.19,58.9
  Bottom 0.254: 119.25,58.9 117.35,56.99 114.81,56.99 104.14,67.66
  Bottom 0.305: v123.19,58.9 119.25,58.9 | 104.14,67.66 CONN4.4
D12  (via drill 0.3 pad 0.3)
  Top 0.305: CONN4.5 101.6,78.33 CONN3.5 | U1.26 112.57,56.69 110.62,58.64 v110.62,60.17
  Bottom 0.305: CONN4.5 102.87,75.41 102.87,67.79 103,67.79 v110.62,60.17
D13
  Top 0.305: CONN3.6 99.06,78.33 CONN4.6 99.06,75.41 100.33,74.14 105.09,74.14 106.05,73.18 106.05,67.79 | U1.32 112.04,51.89 106.05,57.88 106.05,67.79 | R6.1 106.05,67.79
D+  (via drill 0.3 pad 0.3)
  Top 0.254: v123.51,53.5 125.17,53.5 U1.4
  Top 0.305: v28.89,64.93 17.93,75.89 R4.1
  Bottom 0.254: 119.38,55.09 85.72,55.09
  Bottom 0.305: v123.51,53.5 120.97,53.5 119.38,55.09 | 85.72,55.09 79.06,61.75 41.59,61.75 38.42,64.93 v28.89,64.93
D-  (via drill 0.3 pad 0.3)
  Top 0.305: U1.3 v122.87,52.69 | 18,80.8 arc90 R5.1 18.19,80.49 20.32,80.49 v36.83,63.98
  Bottom 0.254: 119.06,54.45 85.41,54.45 | 78.74,61.12 41.27,61.12
  Bottom 0.305: v122.87,52.69 120.83,52.69 119.06,54.45 | 85.41,54.45 78.74,61.12 | 41.27,61.12 38.42,63.98 v36.83,63.98
ECHO  (via drill 0.3 pad 0.3)
  Top 0.305: ULTRASONIC.2 74.93,53.82 v66.04,44.93 | v56.83,46.2 56.83,49.27 U2.37
  Bottom 0.305: v66.04,44.93 58.42,44.93 v56.83,46.2
GND  (via drill 0.3, 0.3 pad 0.3)  (1 unrouted)
  Top 0.254: 114.3,46.2 116.18,48.08 U1.35 116.18,50.3 116.84,50.96 122.24,50.96 122.56,50.64 122.56,49.31 U1.43 122.58,50.67 v122.87,50.96 | C12.2 111.76,42.52 111.76,44.8 | U1.5 126.53,54.29 127,53.82 v127,52.86 128.91,50.96 C3.2 | U1.15 120.98,62.4 v121.92,63.34 | U3.2 v58.74,22.38 | v105.41,75.41 v100.33,75.41 | v60.8,66.99 60.96,66.83 60.96,63.98 60.02,63.04 U2.15 60.01,60.87 60.01,59.85 59.24,59.09 U2.23 | U2.35 55.22,50.62 55.56,50.96 61.28,50.96 61.59,50.64 61.59,49.31 U2.43 61.59,49.26 v61.59,47.47 61.59,43.02 v62.87,41.75 | U2.5 65.57,54.29 66.04,53.82 66.04,53.18 v66.67,52.55 | 32.72,23.04 33.02,23.34 | U5.2 20,33.18 20.32,33.5
  Top 0.305: v113.67,60.8 114.3,60.17 | 111.76,44.8 C10.2 114.3,46.2
  Top 0.406: U4.2 32.72,23.04
  Bottom 0.254: v122.87,50.96 124.14,50.96 124.46,51.28 | v127,52.86 127,53.82 | v62.87,41.75 63.5,41.12
  other vias: 100.01,44.29 57.15,52.7 113.03,69.06 114.3,76.68 97.79,75.41 87.63,65.25 88.9,66.52 90.17,67.79 90.17,65.25 92.71,65.25 91.44,66.52 74.93,30.64 81.28,30.64 90.17,30.64 93.66,36.35 86.36,38.58 86.36,39.85 87.63,41.12 88.9,39.85 88.9,38.58 83.82,38.58 83.82,39.85 85.09,41.12 65.41,43.02 97.79,30.64 97.79,25.56 88.9,25.56 61.28,37.31 51.44,41.75 50.01,44.61 48.26,47.47 63.34,68.58 70.33,65.56 92.71,70.33 93.98,71.6 91.44,71.6 95.25,72.87 90.17,72.87 92.71,72.87 88.9,58.9 83.82,48.1 92.08,50.64 90.81,50.32 92.08,49.05 91.44,49.69 92.71,50.01 68.58,25.88 68.26,20.8 68.26,21.75 59.69,22.38 68.42,68.42 58.9,72.07 57.94,72.07 59.85,72.07 62.55,50.96 69.85,52.23 68.26,51.91 23.81,29.69 33.66,23.34 35.56,23.34 34.61,22.38 33.66,21.43 35.56,21.43 25.08,29.69 23.5,23.65 23.5,25.24 40.96,41.43 40.96,40.16 40.96,38.89 48.26,48.74 49.21,49.69 104.3,57.15 106.36,48.74 106.36,53.02 68.42,70.96 68.42,73.5 68.42,76.04 65.88,78.58 70.96,76.04 70.96,73.5 73.5,76.04 68.42,78.58 65.88,81.12 76.04,76.04 76.04,78.58 73.5,78.58 51.12,76.52 51.12,78.74 48.9,78.74 44.13,70.33 41.75,70.33 39.21,70.33 27.94,79.22 30.48,76.68 33.02,74.14 35.56,71.6 15.24,74.14 17.78,63.98 15.24,63.98 5.08,61.44 7.62,61.44 5.08,58.9 7.62,58.9 17.78,20.8 17.78,23.34 17.78,25.88 17.78,28.42 28.42,48.74 28.42,46.2 32.38,46.99 32.38,49.53 71.6,43.66 71.6,46.2 71.6,41.12 53.82,36.04 51.28,36.04 51.28,33.5 53.82,33.5 110.97,68.26
  pour Top (isolate 0.61): -1.27,105.89 156.21,103.35 156.21,8.1 -1.27,4.29
  pour Bottom (isolate 0.61): 77.47,103.35 77.47,88.11 142.24,88.11 149.86,81.76 156.21,81.76 156.21,29.69 149.86,29.69 142.24,22.07 77.47,22.07 77.47,6.83 35.56,6.83 35.56,18.26 0,18.26 0,91.92 35.56,91.92 35.56,103.35
IR
  Top 0.305: U$10.1 24.13,60.17 38.5,60.17 39.45,59.21 49.93,59.21 51.65,57.49 U2.25
IR_GND  (via drill 0.3)
  Top 0.203: MUX.8 102.87,6.57 102.87,14.61 JP4.6
  Top 0.254: MUX.6 100.97,5.3 v100.97,6.83
  Top 0.305: MUX.8 MUX.7 MUX.6
  Bottom 0.305: Q2.4 84.31,7.73 Q2.2 88,7.73 89.8,5.93 Q3.4 93.19,7.73 Q3.2 96.25,7.73 98.06,5.93 Q4.4 100.06,5.93 v100.97,6.83 101.86,7.73 Q4.2 104.51,7.73 106.31,5.93 Q5.4 109.7,7.73 Q5.2
IR_OUT  (via drill 0.3 pad 0.3)
  Top 0.305: MUX.3 95.25,4.29 95.57,3.97 102.87,3.97 103.98,5.08 v103.98,13.89
  Bottom 0.203: JP4.4 98.42,16.51 101.92,16.51 103.98,14.45 v103.98,13.89
IR_VCC  (via drill 0.3 pad 0.3)
  Top 0.305: MUX.16 v92.71,12.38
  Bottom 0.305: 85.72,10.79 R1.2 | 97.95,1.27 104.3,1.27 106.44,3.41 R15.2 | 97.95,1.27 89.53,1.27 | 89.53,1.27 83.74,1.27 83.03,1.98 R3.2 81.52,3.41 80.64,4.29 80.64,11.27 81.68,12.3 84.93,12.3 85.88,11.36 R1.2 | R11.2 89.93,3.41 89.53,3.02 89.53,1.27 | R13.2 98.35,3.41 97.95,3.02 97.95,1.27 | v92.71,12.38 92.87,12.54 | R1.2 88.02,12.38 v92.71,12.38 | R14.2 111.28,11.04 110.97,11.35 102.23,11.35 | 102.23,11.35 94.61,11.35 | 94.61,11.35 93.74,11.35 v92.71,12.38 | R10.2 94.77,11.2 94.61,11.35 | R12.2 102.39,11.2 102.23,11.35 | JP4.2 92.71,15.88 v92.71,12.38
IRA
  Top 0.203: JP4.1 96.84,13.02 98.19,13.02 99.06,12.14 MUX.11
IRB
  Top 0.203: JP4.3 100.33,12.07 MUX.10
IRC
  Top 0.203: JP4.5 101.6,13.34 MUX.9
MISO
  Top 0.254: JP3.1 134.42,59.09 U1.11
MOSI
  Top 0.203: U1.10 132.69,58.29 133.35,57.63 135.89,57.63 135.89,57.62 JP3.4
MUX0  (via drill 0.3 pad 0.3)
  Top 0.305: v87.63,3.02 87,3.65 87,12.14 88.5,13.65 94.85,13.65 96.52,11.99 MUX.13
  Bottom 0.305: R3.1 86.41,3.54 Q2.3 86.36,5.88 86.36,2.7 86.68,3.02 v87.63,3.02
MUX1  (via drill 0.3 pad 0.3)
  Top 0.305: v96.68,2.22 91.28,2.22 88.58,4.92 88.58,12.38 89.3,13.1 94.38,13.1 95.25,12.22 MUX.14
  Bottom 0.305: 95.25,5.88 Q3.3 95.3,3.54 R11.1 95.81,3.02 v96.68,2.22
MUX2  (via drill 0.3 pad 0.3)
  Top 0.305: MUX.15 93.98,8.73 91.52,6.27 91.52,4.13 92.39,3.25 v104.46,3.25
  Bottom 0.305: 102.23,3.02 102.92,3.7 Q4.3 102.92,3.54 R13.1 102.55,3.25 v104.46,3.25
MUX3  (via drill 0.3 pad 0.3)
  Top 0.305: v97.79,12.22 MUX.12
  Bottom 0.305: R15.1 111.81,3.54 Q5.3 112.77,5.93 113.67,6.83 113.67,10.8 111.6,12.86 98.42,12.86 v97.79,12.22
MUX_OUT  (via drill 0.3 pad 0.3)
  Top 0.305: v102.23,37.31 98.42,33.5 92.71,33.5 91.44,32.23 68.58,32.23 60.02,40.79 U2.41
  Bottom 0.254: 110.49,37.31 v102.23,37.31
  Bottom 0.305: JP2.4 146.05,53.82 146.05,52.55 133.35,39.85 113.03,39.85 110.49,37.31
N$1
  Top 0.406: TX.C R8.2
N$2
  Top 0.406: MINIUSB.2 12.7,80.02 13.42,80.74 R5.2
N$3
  Top 0.305: U2.21 55.22,63.37 49.53,69.06
  Top 0.406: SER_CPU2.1 38.73,79.85 49.53,69.06
N$4
  Top 0.305: U2.20 56.02,63.84 48.26,71.6
  Top 0.406: 48.26,71.6 37.47,82.39 SER_CPU2.2
N$5
  Top 0.406: MINIUSB.3 12.7,79.22 13.46,78.45 R4.2
N$6
  Top 0.305: R9.1 113.54,51.12 U1.33
N$7
  Top 0.406: D13.A R6.2
N$8
  Top 0.305: U2.6 66.04,55.09 66.99,54.13 C9.1
N$9
  Top 0.406: R7.2 RX.C
N$10
  Bottom 0.305: Q2.1 83.03,8.25 R1.1
N$11
  Bottom 0.305: Q3.1 91.92,8.25 R10.1
N$12
  Bottom 0.305: Q4.1 99.54,8.25 R12.1
N$13
  Top 0.406: MINIUSB.1 11.76,80.82 12.7,81.76 12.7,83.03 13.34,83.66 F2.1
N$14
  Bottom 0.305: Q5.1 108.43,8.25 R14.1
N$15
  Top 0.305: U1.6 128.4,55.09 128.91,54.58 C3.1
N$16
  Top 0.305: R18.2 146.47,47.74 FET1.1
N$17
  Top 0.305: U2.33 52.62,45.48 48.9,41.75 R24.1
N$18
  Top 0.406: F1.1 13.34,46.83 12.7,46.2 12.7,45.18 11.51,43.99 MINIUSB1.1
N$19
  Top 0.305: U4.1
  Top 0.406: FET3.1 21.91,22.06 22.54,21.43 27.94,21.43 28.89,22.38 U4.1
N$20
  Top 0.305: U5.5 14.61,32.23 13.34,30.96 13.34,29.69 12.7,29.05 R19.1
N$21
  Top 0.305: U5.1 17.46,32.23 16.51,33.18 13.65,33.18 12.7,32.23 R17.1
N$22
  Top 0.305: D4.C R17.2
N$23
  Top 0.305: 32.07,26.99 R51.2
  Top 0.406: U4.4 31.48,24.34 32.07,24.92 32.07,26.99 | R51.2 31.92,28.58 32.38,29.05 34.61,29.05 34.92,29.37 R49.1
N$24
  Top 0.305: 25.53,36.51 L2.2 25.4,36.54
  Top 0.406: D3.A 25.53,36.51 | FET3.3 23.86,33.54 25.4,35.08 25.4,36.54
N$25
  Top 0.305: 26.94,24.34 26.67,24.34 26.8,24.47
  Top 0.406: U4.8 27.62,22.39 28.26,23.02 | 28.26,23.02 28.93,23.69 U4.3 | U4.5 26.67,24.34 | 26.94,24.34 28.26,23.02 | 26.8,24.47 C19.1 28.89,27.15 31.11,29.37 R46.1
N$26
  Top 0.254: STEPPER_DRIVER.11 85.72,60.8 86.36,61.44 86.36,65.25 X2.P$4
N$27
  Top 0.254: STEPPER_DRIVER.12 81.92,59.53 81.28,60.17 81.28,67.79 X2.P$3
N$28
  Top 0.254: STEPPER_DRIVER.13 81.92,58.26 80.01,60.17 80.01,66.52 X2.P$2
N$29
  Top 0.254: STEPPER_DRIVER.14 81.92,56.99 78.74,60.17 X2.P$1
N$30
  Top 0.254: STEPPER_DRIVER.15 81.92,55.72 80.64,54.45 80.64,44.29 X1.P$4
N$31
  Top 0.254: STEPPER_DRIVER.16 81.92,54.45 81.28,53.82 81.28,42.39 X1.P$3
N$32
  Top 0.254: STEPPER_DRIVER.17 82.23,53.18 81.92,52.86 81.92,40.48 X1.P$2
N$33
  Top 0.254: X1.P$1 80.01,34.77 82.55,37.31 82.55,45.24 86.04,48.74 86.04,50.96 85.09,51.91 STEPPER_DRIVER.18
N$34
  Top 0.305: R20.2 43.03,46.75 D13_2.A
N$35
  Top 0.406: TX1.C R22.2
N$36
  Top 0.406: RX1.C R21.2
N$37
  Top 0.305: MINIUSB1.2 12.74,43.19 13.59,44.04 R25.2
N$38
  Top 0.305: MINIUSB1.3 12.7,42.39 13.59,41.5 R16.2
N$41  (via drill 0.3 pad 0.3)
  Top 0.305: SHIFT2.15 v100.01,46.83
  Bottom 0.254: 110.49,36.35 101.28,36.35 99.06,38.58
  Bottom 0.305: JP2.1 148.59,51.28 145.73,51.28 133.67,39.21 113.35,39.21 110.49,36.35 | v100.01,46.83 99.06,45.88 99.06,38.58
N$42  (via drill 0.3 pad 0.3)
  Top 0.305: v97.79,48.1 SHIFT2.1
  Bottom 0.254: 110.81,35.72 100.97,35.72 98.5,38.18 98.5,47.39 v97.79,48.1
  Bottom 0.305: JP2.3 153.03,54.45 153.03,53.18 150.5,50.64 146.05,50.64 133.99,38.58 113.67,38.58 110.81,35.72
N$43  (via drill 0.3 pad 0.3)
  Top 0.305: v151.76,50.64 153.03,51.91 153.03,57.94 152.08,58.9 JP2.5 | SHIFT2.2 v97.79,46.83
  Bottom 0.254: 111.12,34.77 100.33,34.77 97.79,37.31
  Bottom 0.305: 111.12,34.77 113.98,37.62 134.3,37.62 146.69,50.01 151.13,50.01 v151.76,50.64 | v97.79,46.83 97.79,37.31
N$44  (via drill 0.3 pad 0.3)
  other vias: 133.35,77.95
N$45
  Top 0.254: FET1.3 149.86,57.63 JP2.6
NRF_CE  (via drill 0.3 pad 0.3)
  Top 0.305: v47.78,52.07 50,54.29 U2.29
  Bottom 0.305: U$5.P$2 38.73,22.7 38.73,43.02 v47.78,52.07
NRF_CSN  (via drill 0.3 pad 0.3)
  Top 0.305: v49.05,52.07 50.47,53.49 U2.30
  Bottom 0.305: U$5.P$7 42.23,21.75 42.23,24.29 39.37,27.15 39.37,42.39 v49.05,52.07
NRF_IRQ  (via drill 0.3 pad 0.3)
  Top 0.305: U$5.P$5 47.5,19.53 v49.53,19.53 | v67.31,50.01 66.23,51.09 U2.1
  Bottom 0.305: v67.31,50.01 67.31,36.67 61.91,30.96 58.74,30.96 56.83,29.05 56.83,26.83 v49.53,19.53
RESET  (via drill 0.3 pad 0.3)
  Top 0.305: U1.13 122.58,62.1 123.19,62.71 125.73,62.71 v127,61.44 | v133.22,55.09 133.34,55.09 JP3.5 133.99,53.18 S2.3 v133.99,46.83 S2.4 133.99,41.5 133.45,40.96 R2.1 | v108.46,39.85 108.46,34 107.95,33.5 105.41,33.5 104.14,32.23 CONN5.1
  Bottom 0.305: v127,61.44 130.18,58.26 130.18,55.85 130.94,55.09 v133.22,55.09 | v133.99,46.83 124.21,46.83 119.76,42.39 111,42.39 v108.46,39.85
RX-I
  Top 0.305: CONN2.1 134.62,76.68 132.08,74.14 123.19,74.14 116.98,67.93 U1.20
RXLED  (via drill 0.3 pad 0.3)
  Top 0.305: U1.8 122.89,56.69 v122.87,56.67 | v13.97,69.06 R7.1 11.43,69.06
  Bottom 0.254: 119.38,55.72 86.04,55.72
  Bottom 0.305: v122.87,56.67 120.33,56.67 119.38,55.72 | 86.04,55.72 79.38,62.39 42.23,62.39 38.1,66.52 19.05,66.52 16.51,69.06 v13.97,69.06
S1
  Top 0.406: SHIFT1.15 100.33,58.26 97.79,60.8 STEPPER_DRIVER.8
S1OVERFLOW
  Top 0.305: SHIFT2.14 103.5,45.56 104.14,46.2 104.14,50.01 103.5,50.64 SHIFT1.9
S2
  Top 0.406: SHIFT1.1 STEPPER_DRIVER.7
S2O4  (via drill 0.3 pad 0.3)
  Top 0.305: v139.7,41.12 139.7,46.2 140.97,47.47 R18.1 | v94.3,45.56 SHIFT2.3
  Bottom 0.254: 111.44,33.81 100.01,33.81 93.34,40.48
  Bottom 0.305: v139.7,41.12 135.25,36.67 114.3,36.67 111.44,33.81 | 93.34,40.48 93.34,44.61 v94.3,45.56
S3
  Top 0.406: SHIFT1.2 STEPPER_DRIVER.6
S4
  Top 0.406: STEPPER_DRIVER.5 SHIFT1.3
S5
  Top 0.406: STEPPER_DRIVER.4 SHIFT1.4
S6
  Top 0.406: STEPPER_DRIVER.3 SHIFT1.5
S7
  Top 0.406: STEPPER_DRIVER.2 SHIFT1.6
S8
  Top 0.406: STEPPER_DRIVER.1 SHIFT1.7
S_GRIP  (via drill 0.3 pad 0.3)
  Top 0.305: v89.22,81.44 90.49,82.71 134.62,82.71 140.65,76.68 SERVO2(GRIP).3 | v87.63,79.85 85.09,79.85 v80.33,75.09 | v48.9,65.25 48.26,64.61 v48.26,60.17 | U2.27 48.73,55.89 48.26,56.36 v48.26,57.63
  Bottom 0.305: v89.22,81.44 v87.63,79.85 | v80.33,75.09 79.38,74.14 76.2,74.14 68.58,66.52 62.23,66.52 60.96,65.25 v48.9,65.25 | v48.26,57.63 v48.26,60.17
S_GRIPROT  (via drill 0.3 pad 0.3)
  Top 0.305: U2.12 65.32,60.89 v68.58,57.63
  Bottom 0.254: 111.76,33.18 99.69,33.18 92.71,40.16
  Bottom 0.305: SERVO3(GRIPROT).3 138.43,38.58 135.89,36.04 114.62,36.04 111.76,33.18 | 92.71,40.16 92.71,46.2 87.63,51.28 85.09,51.28 | 82.55,48.74 76.2,48.74 73.66,51.28 73.66,55.09 71.12,57.63 v68.58,57.63
  Bottom 0.406: 85.09,51.28 82.55,48.74
S_USONIC  (via drill 0.3 pad 0.3)
  Top 0.305: v101.44,38.1 97.47,34.13 92.08,34.13 91.12,33.18 68.9,33.18 v60.96,41.12 | v54.61,52.55 54.47,52.69 U2.31
  Bottom 0.254: 110.33,38.1 v101.44,38.1
  Bottom 0.305: SERVO1(USONIC).3 141.6,58.9 140.97,58.26 140.97,48.42 133.03,40.48 112.71,40.48 110.33,38.1 | v60.96,41.12 58.42,41.12 54.61,44.93 v54.61,52.55
SCK
  Top 0.305: JP3.3 133.35,56.36 132.22,57.49 U1.9
SCL  (via drill 0.3 pad 0.3)
  Top 0.305: CONN3.10 88.9,78.33 CONN4.10 | U1.18 v118.58,67.37 | CONN3.10 91.57,80.99 126.11,80.99 127,80.11 CONN2.4 | CONN3.10 87.25,81.76 79.38,81.76 78.74,82.39 R26.1 78.74,84.3 78.11,84.93 69.22,84.93 U$4.P$3 | U2.18 57.62,64.78 45.72,76.68 U$3.P$3
  Bottom 0.305: CONN2.4 127,75.79 v118.58,67.37 | U$4.P$3 66.04,88.11 46.99,88.11 U$3.P$3
SD_CS  (via drill 0.3 pad 0.3)
  Top 0.305: v46.99,64.61 v46.99,60.17 | v46.99,57.63 46.99,56.36 48.26,55.09 U2.28
  Bottom 0.305: U$2.P$9 53.37,71.57 54.61,70.33 54.61,67.79 53.34,66.52 48.26,66.52 46.99,65.25 v46.99,64.61 | v46.99,60.17 v46.99,57.63
SDA  (via drill 0.3 pad 0.3)
  Top 0.305: U1.19 v117.78,64.99 | CONN3.9 91.44,78.33 CONN4.9 | v88.91,83.18 R27.1 82.55,84.3 81.28,85.57 71.12,85.57 U$4.P$4 68.58,88.11 49.53,88.11 U$3.P$4 46.99,85.57 v46.99,83.03 | U2.19 56.82,64.31 v53.34,67.79
  Bottom 0.305: v117.78,64.99 117.86,64.99 129.54,76.68 CONN2.3 129.54,81.12 128.27,82.39 115.32,82.39 113.92,80.99 94.11,80.99 CONN3.9 92.39,79.28 92.39,82.87 92.08,83.18 v88.91,83.18 | v53.34,67.79 53.34,70.33 46.99,76.68 v46.99,83.03
SHIFT_RCK  (via drill 0.3 pad 0.3)
  Top 0.305: SHIFT1.12 104.14,54.45 104.78,53.82 104.78,43.66 104.14,43.02 SHIFT2.12 100.65,43.02 100.33,42.7 v100.33,41.75 | U2.26 50.47,56.69 48.58,58.58 45.72,58.58 44.45,57.31 44.45,31.27 45.72,30 v45.72,26.51 | v48.9,21.43 50.16,21.43 53.34,18.26 68.58,18.26 v77.47,27.15 | v100.33,39.21 v96.2,35.08
  Bottom 0.305: v45.72,26.51 45.72,24.61 v48.9,21.43 | v100.33,41.75 v100.33,39.21 | v96.2,35.08 93.98,32.86 93.98,28.42 92.71,27.15 v77.47,27.15
TFT_CS  (via drill 0.3 pad 0.3)
  Top 0.305: U2.40 v59.22,33.66
  Bottom 0.305: v59.22,33.66 58.74,33.18 57.15,33.18 52.95,28.98 U$2.P$3
TFT_DC
  Top 0.305: U2.38 57.62,31.12 58.1,30.64 58.1,28.54 U$2.P$5
TFT_RST  (via drill 0.3 pad 0.3)
  Top 0.305: U2.39 v58.42,32.23
  Bottom 0.305: v58.42,32.23 55.49,29.3 U$2.P$4
TRIG  (via drill 0.3 pad 0.3)
  Top 0.305: ULTRASONIC.3 76.2,56.36 v63.5,43.66 | v56.2,45.24 56.02,45.42 U2.36
  Bottom 0.305: v63.5,43.66 57.78,43.66 v56.2,45.24
TX-O
  Top 0.305: CONN2.2 132.08,76.68 130.81,75.41 123.19,75.41 116.18,68.4 U1.21
TXLED  (via drill 0.3 pad 0.3, 0.6)
  Top 0.254: v119.38,56.99 119.38,57.63
  Top 0.305: U1.22 115.38,59.4 115.57,59.21 117.79,59.21 119.38,57.63 | v19.21,69.06 17.78,69.06 14.61,65.88 R8.1
  Bottom 0.254: 86.36,56.36 118.75,56.36 v119.38,56.99
  Bottom 0.305: 86.36,56.36 79.69,63.02 42.55,63.02 38.42,67.15 21.11,67.15 v19.21,69.06
USB_VIN  (via drill 0.3, 0.6)
  Top 0.406: C20.1 2.31,29.05 D4.A 4.21,34.13 U5.4 v14.29,34.13 | v19.84,46.83 C5.1 F1.2 | F2.2 v20.8,83.66 C6.1
  Bottom 0.406: v14.29,34.13 16.51,36.35 16.51,44.61 18.73,46.83 v19.84,46.83 20.95,46.83 23.97,49.85 23.97,55.07 SW1.3 23.5,60.64 11.43,60.64 8.73,63.34 8.73,71.6 v20.8,83.66
VBATT  (via drill 0.3 pad 0.3)  (1 unrouted)
  Top 0.305: 11.56,21.56 C18.2 | 17.46,34.13 U5.3
  Top 0.406: 5.12,20.8 10.79,20.8 11.56,21.56 | C18.2 C21.1 12.7,25.88 14.61,27.78 14.61,30.32 15.24,30.96 v15.88,30.96 | v16.83,34.13 17.46,34.13 | U5.3 19.68,34.13 20.32,34.77 20.32,36.04 20.95,36.67 L2.1 | BATT.2 3.94,21.94 5.08,20.8
  Bottom 0.406: v15.88,30.96 16.83,31.91 v16.83,34.13
VCC  (via drill 0.3, 0.3 pad 0.3)  (1 unrouted)
  Top 0.305: U1.7 125.22,55.85 | 131.44,54.58 C4.1 | 110.36,46.07 110.49,46.2 | 110.49,46.33 C10.1 | RX1.A TX.A | U3.1 55.88,23.34 | 62.23,85.57 U$4.P$1 | SHIFT1.10 100.01,51.91 99.06,50.96 99.06,48.1 | 99.06,48.1 99.06,41.12 99.69,40.48 SHIFT2.10 | SHIFT2.16 99.06,48.1 | JP2.2 146.05,56.36 146.69,56.99 | v45.85,37.44 45.72,37.31 | TX1.A 2.31,51.51 3.81,50.01 19.05,50.01 U$10.3
  Top 0.406: TX.A RX.A | 131.44,54.58 130.18,55.85 125.22,55.85 121.78,55.85 | 121.78,51.89 116.81,51.89 115.38,50.45 U1.34 112.31,49.29 v111.76,48.74 110.49,47.47 110.49,46.33 | 121.78,51.89 U1.2 126.39,51.89 127,51.28 127,49.37 130.81,45.56 R2.2 | U1.14 121.78,55.85 | 121.78,55.85 121.78,51.89 | v131.44,56.36 C4.1 | 110.36,46.07 L1.1 C12.1 110.36,33.37 109.22,32.23 CONN5.3 | RX1.A TX1.A | U3.1 51.76,23.33 47.87,27.22 U$2.P$1 47.87,30.08 45.85,32.1 45.85,35.14 | 55.88,23.34 55.88,21.43 U3.3 | R26.2 R27.2 | R26.2 X2.P$5 | R26.2 76.35,80.33 72.39,84.3 63.5,84.3 62.23,85.57 | X1.P$5 80.01,46.2 80.01,57.94 79.06,58.9 ULTRASONIC.4 75.88,58.9 | 75.88,58.9 75.25,59.53 75.25,62.39 76.83,63.98 76.83,73.5 X2.P$5 | SHIFT2.10 104.14,40.48 106.36,42.7 v106.36,46.2 | JP3.2 139.69,56.36 SERVO1(USONIC).2 146.05,56.36 | SERVO3(GRIPROT).2 145.41,36.04 146.05,36.67 146.05,43.66 144.78,44.93 144.78,50.01 JP2.2 | 146.69,56.99 146.69,72.87 145.41,74.14 SERVO2(GRIP).2 | 60.82,51.89 55.54,51.89 54.42,50.77 U2.34 54.42,41.88 51.75,39.21 C2.1 v45.85,37.44 45.85,36.04 45.85,35.14 | 60.82,51.89 U2.2 | U2.14 60.82,55.89 | 60.82,55.89 60.82,51.89 | 60.82,55.89 U2.7 72.87,55.89 75.88,58.9 | SHIFT1.16 100.33,59.53 v98.42,61.44 86.36,73.5 80.64,73.5 X2.P$5 | STEPPER_DRIVER.10 v85.09,62.07 | U$10.3 23.94,52.55 SW1.2 30.48,51.15 v30.48,50.01 30.48,42.23 34.45,38.26 38.1,38.26 | 38.1,38.26 38.26,38.26 39.21,37.31 v41.91,37.31 | R23.2 38.1,40.79 38.1,38.26 | C17.1 45.85,35.14
  Bottom 0.254: JP1.2 35.56,56.36 33.02,56.36 30.48,53.82
  Bottom 0.305: 30.48,53.82 v30.48,50.01 | 45.72,37.31 v45.85,37.44
  Bottom 0.406: JP3.2 135.25,60.8 132.72,60.8 131.44,59.53 v131.44,56.36 | U$4.P$1 62.23,85.57 61.59,84.93 41.27,84.93 40.64,85.57 U$3.P$1 | v106.36,46.2 108.9,48.74 v111.76,48.74 | X2.P$5 87.63,84.3 135.89,84.3 140.97,79.22 140.97,74.61 141.45,74.14 SERVO2(GRIP).2 | v41.91,37.31 45.72,37.31 | v85.09,62.07 97.79,62.07 v98.42,61.44
XTAL1
  Top 0.406: Q1.1 124.21,70.33 | 124.21,70.33 C15.1 | U1.17 119.38,66.9 122.81,70.33 124.21,70.33
XTAL2
  Top 0.406: C16.1 124.21,66.52 Q1.2 123.81,65.25 121.92,65.25 120.18,63.51 U1.16

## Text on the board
Top: EDUBOT V0.12 BY / SEBASTIAN MUSZYTOWSKI | USER

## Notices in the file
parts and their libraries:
SparkFun-Connectors: Licensing: Creative Commons ShareAlike 4.0 International - https://creativecommons.org/licenses/by-sa/4.0
